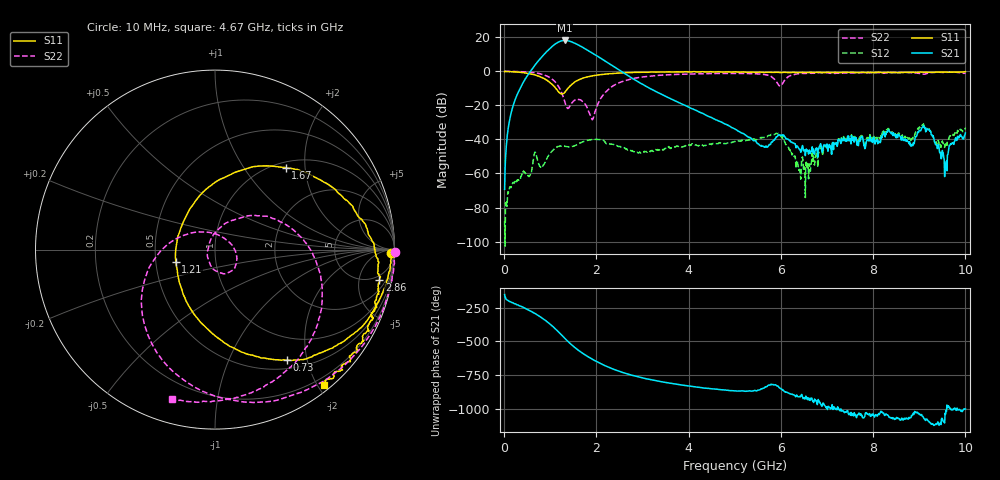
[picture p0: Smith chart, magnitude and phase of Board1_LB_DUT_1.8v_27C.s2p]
! Created Tue May 27 15:26:42 2025
# hz S ma R 50
! 2 Port Network Data from SP1.SP block
! freq  magS11  angS11  magS21  angS21  magS12  angS12  magS22  angS22
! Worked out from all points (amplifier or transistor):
!   1000 points, 10 MHz to 10 GHz, reference 50 ohm
!   highest |S21| = 18.1 dB at 1.31 GHz (marker M1)
!   |S21| within 3 dB of that: 1.063 GHz to 1.634 GHz (570.5 MHz wide, 42.3 % of centre)
!   unconditionally stable (mu >= 1): 57.64 MHz to 63.88 MHz; 89.86 MHz to 108.3 MHz; 111.9 MHz to end of sweep
!   at 1.67 GHz: K = 7.31, MAG = 16.6 dB, |S12| = -41.9 dB
!   at 5.01 GHz: K = 43.40, MAG = -15.7 dB, |S12| = -41.2 dB
!   at 10 GHz: K = 15.35, MAG = -16.4 dB, |S12| = -33.1 dB
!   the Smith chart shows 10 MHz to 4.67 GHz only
!   S11 on the Smith chart (normalised r, x): 10 MHz: 59, -52; 730 MHz: 0.62, -1.67; 1.21 GHz: 0.64, -0.09; 1.67 GHz: 1.10, +1.58; 2.86 GHz: 4, -9; 4.67 GHz: 0.09, -2.09
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1e7  0.9811 -1.0  0.0003421 -151.5  3.956e-05 126.3  1.005 -0.8
1.9e8  0.968 -12.9  0.09358 147.8  0.0005373 79.4  0.995 -17.0
7.3e8  0.7357 -57.0  1.949 54.9  0.002312 59.2  0.8783 -75.9
9e8  0.5756 -77.0  3.525 15.0  0.002437 111.8  0.7538 -102.2
1.04e9  0.4128 -101.2  5.379 -23.8  0.004594 100.6  0.5897 -130.5
1.13e9  0.3047 -125.7  6.656 -52.5  0.005856 86.9  0.4474 -153.3
1.21e9  0.2283 -163.0  7.572 -79.9  0.00635 74.6  0.3022 -178.8
1.31e9  0.2373 136.5  8.06 -115.0  0.006342 61.9  0.135 133.0
1.46e9  0.4041 82.8  7.351 -164.1  0.006053 59.3  0.1136 -3.7
1.67e9  0.6026 49.3  5.356 139.6  0.00807 53.2  0.1413 -71.5
1.68e9  0.6095 48.1  5.258 137.2  0.008232 52.2  0.1367 -73.9
1.88e9  0.7227 30.7  3.66 94.2  0.009756 33.0  0.0476 -156.5
2.08e9  0.7959 18.6  2.489 57.5  0.009814 10.6  0.1511 70.0
2.42e9  0.8755 3.3  1.254 7.5  0.006679 -8.0  0.4142 20.1
2.86e9  0.9314 -10.6  0.5364 -38.9  0.00414 -3.9  0.6378 -20.5
3.34e9  0.9521 -23.3  0.2348 -74.8  0.004803 10.1  0.7589 -51.0
4.67e9  0.9671 -51.1  0.03391 -137.3  0.007941 -4.6  0.8638 -106.1
5.01e9  0.9683 -57.8  0.02005 -146.7  0.008675 -9.1  0.8682 -118.0
6.67e9  0.9322 -89.9  0.004963 159.2  0.002621 163.1  0.8787 -149.0
8.34e9  0.9245 -136.2  0.01887 20.6  0.02053 29.6  0.9025 172.3
9.57e9  0.9487 -168.9  0.001353 38.9  0.006993 55.8  0.9239 162.3
1e10  0.9742 177.4  0.01546 78.6  0.02212 71.0  0.8975 156.0
